FUNCTION_BLOCK Axis_PTP IMPLEMENTS ITF_Axis
VAR_INPUT
	DrvIn:ST_DrvIn;
	PARA:ST_AxisPara;
END_VAR

VAR_OUTPUT	
END_VAR
VAR
	REF: AXIS_REF;
	Status:ST_AxisStatus;	
END_VAR

(*
REF.ReadStatus();
Status.Axis_Ready:=REF.Status.ControlLoopClosed;
Status.Axis_Err:=REF.Status.Error;
Status.Axis_IsPTP:=REF.Status.PTPmode;
Status.Current_Pos:=REF.NcToPlc.ActPos;*)

{warning 'add method implementation'}
METHOD M_MoveVel : BOOL
VAR_INPUT
	Execute	: BOOL;
END_VAR
VAR_STAT
	mcMoveVel: Tc2_MC2.MC_MoveVelocity;
END_VAR
mcMoveVel(
	Axis:= REF, 
	Execute:= Execute, 
	Velocity:= PARA.MoveVelo  );
END_METHOD

{warning 'add method implementation'}
METHOD M_PowerOff : BOOL
VAR_STAT
	mcPower: mc_Power;
END_VAR
mcPower(
	Axis:= REF, 
	Enable:=FALSE , 
	Enable_Positive:=TRUE , 
	Enable_Negative:=TRUE , 
	Override:=PARA.rOverride  );
END_METHOD

{warning 'add method implementation'}
METHOD M_PowerOn : BOOL
VAR_STAT
	mcPower: mc_Power;
END_VAR
mcPower(
	Axis:= REF, 
	Enable:=TRUE , 
	Enable_Positive:=TRUE , 
	Enable_Negative:=TRUE , 
	Override:=PARA.rOverride  );
END_METHOD

{warning 'add method implementation'}
METHOD M_Stop : BOOL
VAR_INPUT
	Execute	: BOOL;
END_VAR
VAR_STAT
	mcStop:Tc2_MC2.MC_Stop;
END_VAR
mcStop(
	Axis:= REF, 
	Execute:=Execute );
END_METHOD

{warning 'add property implementation'}
PROPERTY P_Status : ST_AxisStatus
GET
//Can handle the elments of property structure seperately.
//P_Status.Axis_Ready:=REF.Status.ControlLoopClosed;
//P_Status.Axis_IsPTP:=REF.Status.PTPmode;

P_Status:=Status;  // only for property demo, equal to use Status as output variables.
END_GET
END_PROPERTY

END_FUNCTION_BLOCK
